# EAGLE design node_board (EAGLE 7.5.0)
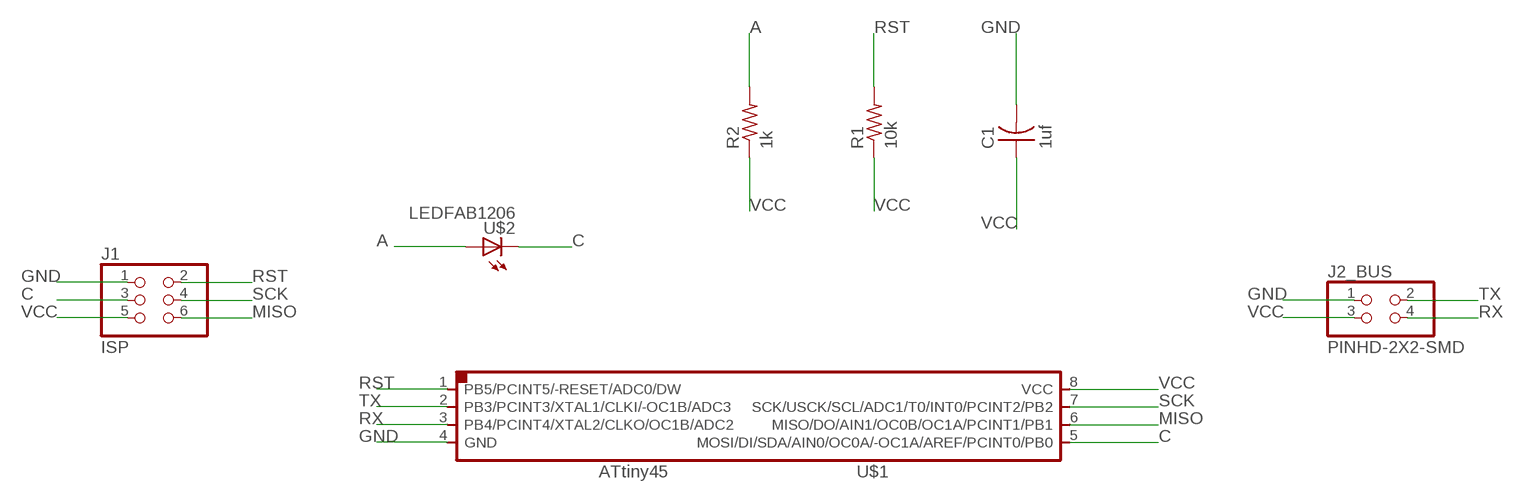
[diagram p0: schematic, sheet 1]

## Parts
C1  1uf  CAP-US1206FAB  [C1206FAB]
J1  ISP  PINHD-2X3-SMD  [2X03SMD]
J2_BUS  PINHD-2X2-SMD  [2X02SMD]
R1  10k  RES-US1206FAB  [R1206FAB]
R2  1k  RES-US1206FAB  [R1206FAB]
U$1  ATTINY45SI  [SOIC8]
U$2  LEDFAB1206  [LED1206FAB]

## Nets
A: R2.2 U$2.1(A)
C: J1.3 U$1.5(MOSI/DI/SDA/AIN0/OC0A/-OC1A/AREF/PCINT0/PB0) U$2.2(C)
GND: C1.2 J1.1 J2_BUS.1 U$1.4(GND)
MISO: J1.6 U$1.6(MISO/DO/AIN1/OC0B/OC1A/PCINT1/PB1)
RST: J1.2 R1.2 U$1.1(PB5/PCINT5/-RESET/ADC0/DW)
RX: J2_BUS.4 U$1.3(PB4/PCINT4/XTAL2/CLKO/OC1B/ADC2)
SCK: J1.4 U$1.7(SCK/USCK/SCL/ADC1/T0/INT0/PCINT2/PB2)
TX: J2_BUS.2 U$1.2(PB3/PCINT3/XTAL1/CLKI/-OC1B/ADC3)
VCC: C1.1 J1.5 J2_BUS.3 R1.1 R2.1 U$1.8(VCC)

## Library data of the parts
C1 = fab:CAP-US
J1 = fab:PINHD-2X3-SMD: PIN HEADER
J2_BUS = fab:PINHD-2X2-SMD
R1 R2 = fab:RES-US: Resistor (US Symbol)
U$1 = fab:ATTINY45
U$2 = fab:LED: LED

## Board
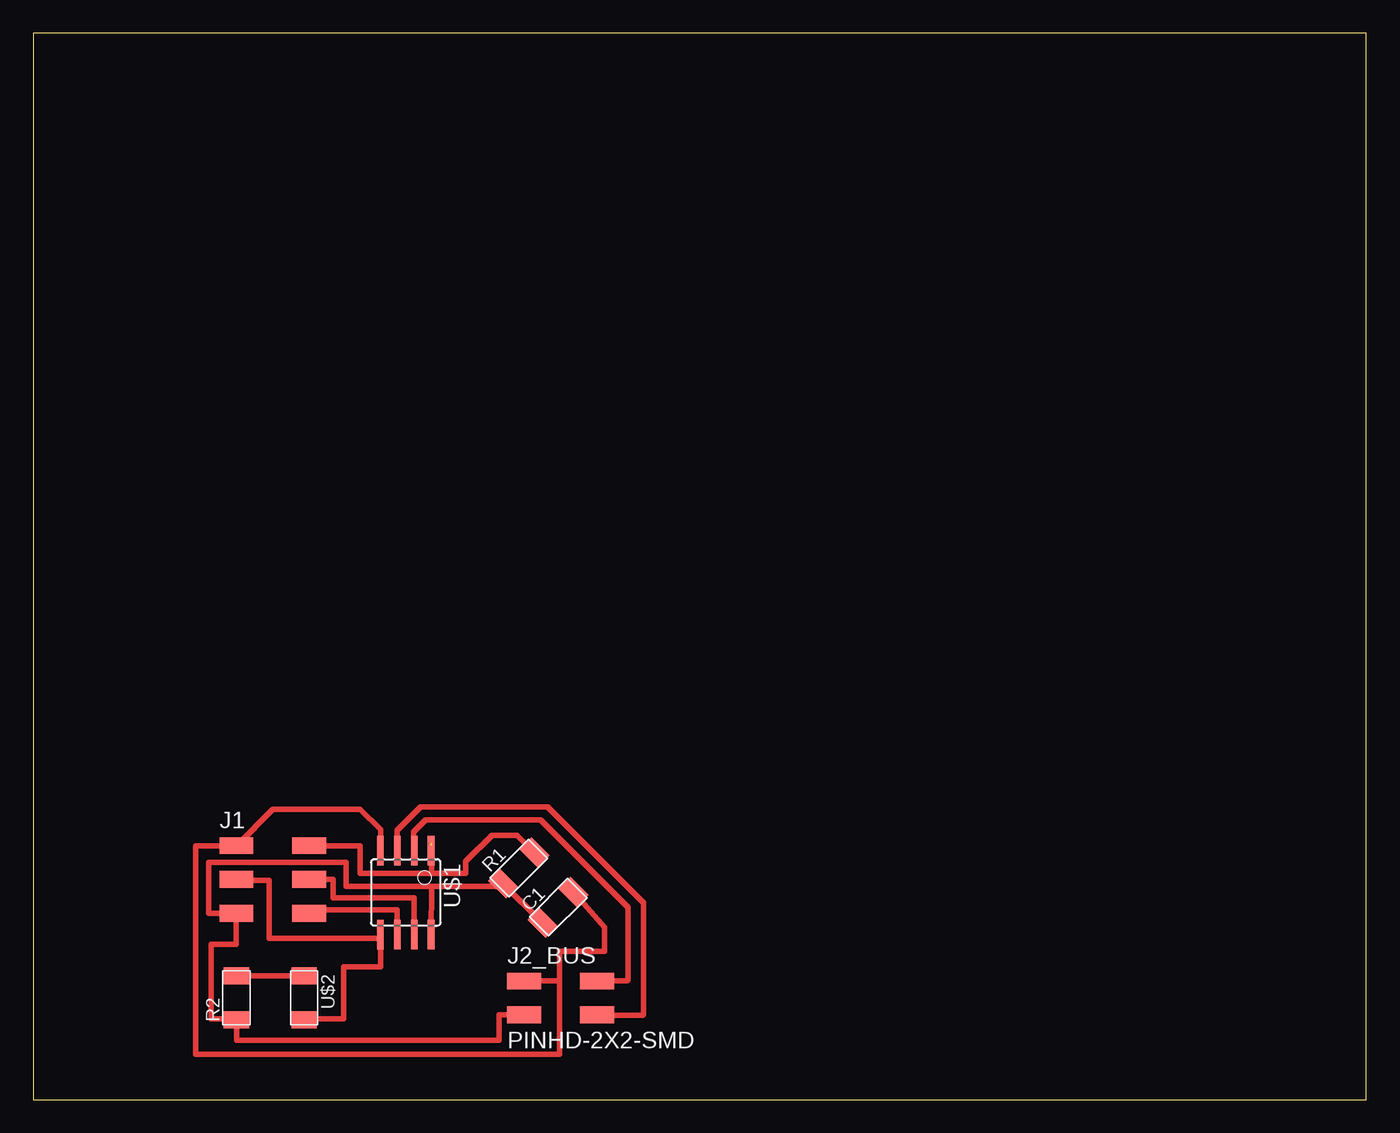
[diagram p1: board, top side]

Size 100 x 80 mm. Coordinates in mm from the lower left corner, seen from the top.
Outline: 0,0 100,0 100,80 0,80 0,0
Copper layers (1*16): Top 0.035mm / dielectric 1.5mm / Bottom 0.035mm
Design rules "default": minimum track width 10mil, minimum drill 24mil, track to track 8mil, track to pad 8mil, pad to pad 8mil, via to via 8mil, smd to smd 8mil, copper to edge 40mil, drill to drill 8mil, minimum pad ring 10mil, minimum via ring 8mil, stop-mask expansion 4mil, vias tented up to drill 0mil, thermal gap 10mil

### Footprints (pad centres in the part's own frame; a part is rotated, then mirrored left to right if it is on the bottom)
C1206FAB = smd 1.27 x 1.905: 1 -1.651,0; 2 1.651,0
2X03SMD = smd 2.54 x 1.27: 1 -2.54,2.54; 2 2.92,2.54; 3 -2.54,0; 4 2.92,0; 5 -2.54,-2.54; 6 2.92,-2.54
2X02SMD = smd 2.54 x 1.27: 1 -2.54,1.27; 2 2.92,1.27; 3 -2.54,-1.27; 4 2.92,-1.27
R1206FAB = smd 1.27 x 1.905: 1 -1.651,0; 2 1.651,0
SOIC8 = smd 0.5 x 2.2: 1 -1.905,-3.154; 2 -0.645,-3.154; 3 0.625,-3.154; 4 1.895,-3.154; 5 1.905,3.154; 6 0.635,3.154; 7 -0.635,3.154; 8 -1.905,3.154
LED1206FAB = smd 1.27 x 1.905: 1 -1.651,0; 2 1.651,0

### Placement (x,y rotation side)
C1  39.37,14.42 45 top
J1  17.78,16.51 0 top
J2_BUS  39.37,7.62 0 top
R1  36.43,17.37 45 top
R2  15.24,7.62 90 top
U$1  27.94,15.53 180 top
U$2  20.32,7.62 270 top

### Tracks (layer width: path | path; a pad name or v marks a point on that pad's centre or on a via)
A
  Top 0.406: U$2.1 R2.2
C
  Top 0.406: U$2.2 20.32,6.04 23.29,6.04 23.29,9.96 26.05,9.96 U$1.5 26.04,12.09 17.69,12.09 17.69,16.45 15.3,16.45 J1.3
GND
  Top 0.406: U$1.4 26.05,20.27 24.54,21.78 17.97,21.78 J1.1 15.24,19.02 12.18,19.02 12.18,3.38 39.47,3.38 39.47,8.89 | 39.47,8.89 39.47,11.11 42.85,11.11 42.85,12.92 C1.2 40.88,15.21 | J2_BUS.1 39.47,8.89
MISO
  Top 0.406: U$1.6 27.29,14.22 20.7,14.22 J1.6
RST  (1 unrouted)
  Top 0.406: U$1.1 29.87,18.69 29.87,19.29 | 37.23,19.24 R1.2 36.3,19.82 34.4,19.82 32.45,17.87 32.45,16.98 29.87,16.98 | 29.87,19.05 29.87,16.98 | J1.2 20.7,19.02 24.54,19.02 24.54,16.98 29.87,16.98
RX
  Top 0.406: U$1.3 27.29,18.69 27.29,20.18 29.07,21.96 38.58,21.96 45.78,14.76 45.78,6.4 45.7,6.31 42.29,6.31 J2_BUS.4
SCK
  Top 0.406: J1.4 22.49,16.51 22.49,15.11 28.57,15.11 U$1.7
TX
  Top 0.406: U$1.2 28.54,18.69 28.54,20.09 29.43,20.98 38.05,20.98 44.63,14.4 44.63,8.98 44.54,8.89 J2_BUS.2
VCC
  Top 0.406: C1.1 R1.1 35.06,16 29.87,16 | J2_BUS.3 34.94,6.35 34.94,4.45 15.24,4.45 R2.1 15.24,6.04 13.34,6.04 13.34,11.65 15.2,11.65 15.2,13.97 J1.5 15.24,13.96 13.16,13.96 13.16,17.78 23.47,17.78 23.47,16 29.87,16 | U$1.8 29.87,16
